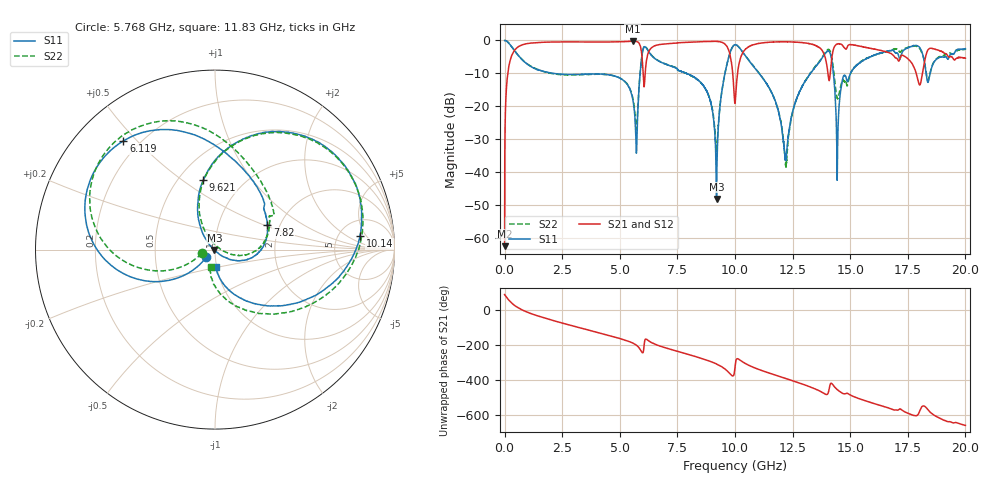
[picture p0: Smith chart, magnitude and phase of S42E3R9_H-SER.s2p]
!{S42E3R9}
!Johanson Technology Inc.
!www.johansontechnology.com
!Test Board Conditions:
!Substrate Type  RO4350B
!Substrate Thickness  50 mil
!Substrate Dk  3.66
!TL Type: GCPW
!TL Trace Width  60 mil
!TL Gap  10 mil
!Electrode orientation  Horizontal
!DUT TOPOLOGY	SERIES
!Mounting Pad LxW  14x55 mil
! Created Wed Nov 25 21:45:00 2020
# khz S ma R 50
! 2 Port Network Data from SP1.SP block
! freq  magS11  angS11  magS21  angS21  magS12  angS12  magS22  angS22
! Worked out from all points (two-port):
!   20001 points, 300 kHz to 20 GHz, reference 50 ohm
!   highest |S21| = -0.24 dB at 5.56 GHz (marker M1); lowest = -62.5 dB at 300 kHz (marker M2)
!   |S21| within 3 dB of the highest: 405 MHz to 5.936 GHz (5.531 GHz wide, 174 % of centre); 6.265 GHz to 9.741 GHz (3.476 GHz wide, 43.4 % of centre)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
!   lowest |S11| = -48.2 dB at 9.198 GHz (marker M3), VSWR 1.01, Z = 49.7 - j0.238 ohm
!   |S11| at or under -10 dB: 2.129 GHz to 5.882 GHz (3.752 GHz wide, 93.7 % of centre); 7.895 GHz to 9.564 GHz (1.669 GHz wide, 19.1 % of centre); 11.04 GHz to 13.27 GHz (2.225 GHz wide, 18.3 % of centre)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
!   |S22| runs from -38.5 to 0.0 dB; largest |S21 - S12| = 0.02
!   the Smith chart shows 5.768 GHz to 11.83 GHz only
!   S11 on the Smith chart (normalised r, x): 5.768 GHz: 0.90, -0.08; 6.119 GHz: 0.14, +0.46; 7.82 GHz: 1.72, +0.53; 9.621 GHz: 0.66, +0.60; 10.14 GHz: 8.01, +3.56; 11.83 GHz: 0.99, -0.19
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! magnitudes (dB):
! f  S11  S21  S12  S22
! 300 kHz  0.0  -62.5  -62.7  0.0
! 120.3 MHz  -0.4  -11.1  -11.1  -0.4
! 389.3 MHz  -2.7  -3.4  -3.4  -2.7
! 3.334 GHz  -10.3  -0.5  -0.5  -10.4
! 5.56 GHz  -17.7  -0.2  -0.2  -17.3
! 5.768 GHz  -23.7  -0.4  -0.4  -22.4
! 6.119 GHz  -2.0  -8.4  -8.4  -1.9
! 6.667 GHz  -6.2  -1.3  -1.3  -6.1
! 7.82 GHz  -9.8  -0.6  -0.6  -9.8
! 8.813 GHz  -16.0  -0.3  -0.3  -16.0
! 9.198 GHz  -48.2  -0.3  -0.3  -33.7
! 9.621 GHz  -8.1  -1.5  -1.6  -8.1
! 10 GHz  -1.3  -19.1  -19.1  -1.3
! 10.14 GHz  -1.8  -8.3  -8.2  -1.8
! 11.83 GHz  -20.2  -0.4  -0.4  -20.2
! 12.21 GHz  -35.9  -0.4  -0.4  -37.7
! 13.33 GHz  -9.5  -1.2  -1.1  -9.3
! 14.1 GHz  -3.5  -12.0  -11.9  -2.9
! 14.45 GHz  -31.6  -1.1  -1.0  -17.7
! 14.73 GHz  -10.7  -2.1  -2.1  -12.4
! 16.67 GHz  -3.2  -3.6  -3.9  -3.2
! 20 GHz  -2.5  -5.4  -5.3  -2.7
